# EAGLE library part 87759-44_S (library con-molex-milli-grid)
HEADER
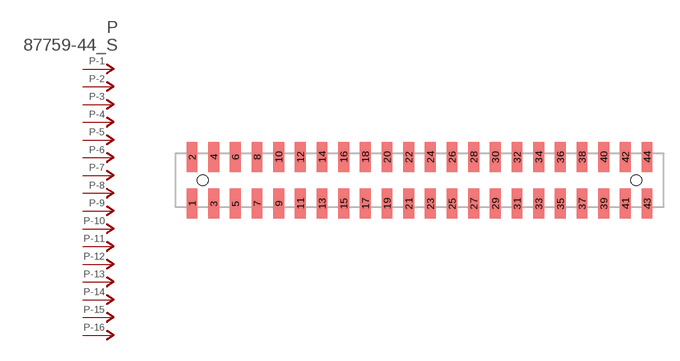
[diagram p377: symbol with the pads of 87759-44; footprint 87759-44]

Designator prefix P; gates -1=P-NV -2=P-N -3=P-N -4=P-N -5=P-N -6=P-N -7=P-N -8=P-N -9=P-N -10=P-N -11=P-N -12=P-N -13=P-N -14=P-N -15=P-N -16=P-N -17=P-N -18=P-N -19=P-N -20=P-N -21=P-N -22=P-N -23=P-N -24=P-N -25=P-N -26=P-N -27=P-N -28=P-N -29=P-N -30=P-N -31=P-N -32=P-N -33=P-N -34=P-N -35=P-N -36=P-N -37=P-N -38=P-N -39=P-N -40=P-N -41=P-N -42=P-N -43=P-N -44=P-N

## 87759-44_S  [87759-44]
1  -1:P  pas
2  -2:P  pas
3  -3:P  pas
4  -4:P  pas
5  -5:P  pas
6  -6:P  pas
7  -7:P  pas
8  -8:P  pas
9  -9:P  pas
10  -10:P  pas
11  -11:P  pas
12  -12:P  pas
13  -13:P  pas
14  -14:P  pas
15  -15:P  pas
16  -16:P  pas
17  -17:P  pas
18  -18:P  pas
19  -19:P  pas
20  -20:P  pas
21  -21:P  pas
22  -22:P  pas
23  -23:P  pas
24  -24:P  pas
25  -25:P  pas
26  -26:P  pas
27  -27:P  pas
28  -28:P  pas
29  -29:P  pas
30  -30:P  pas
31  -31:P  pas
32  -32:P  pas
33  -33:P  pas
34  -34:P  pas
35  -35:P  pas
36  -36:P  pas
37  -37:P  pas
38  -38:P  pas
39  -39:P  pas
40  -40:P  pas
41  -41:P  pas
42  -42:P  pas
43  -43:P  pas
44  -44:P  pas

## Footprint 87759-44 (pad centres in mm)
HEADER SMD Dual Row, Vertical
smd 1 x 2.75: 1 -21,-2.15; 2 -21,2.15; 3 -19,-2.15; 4 -19,2.15; 5 -17,-2.15; 6 -17,2.15; 7 -15,-2.15; 8 -15,2.15; 9 -13,-2.15; 10 -13,2.15; 11 -11,-2.15; 12 -11,2.15; 13 -9,-2.15; 14 -9,2.15; 15 -7,-2.15; 16 -7,2.15; 17 -5,-2.15; 18 -5,2.15; 19 -3,-2.15; 20 -3,2.15; 21 -1,-2.15; 22 -1,2.15; 23 1,-2.15; 24 1,2.15; 25 3,-2.15; 26 3,2.15; 27 5,-2.15; 28 5,2.15; 29 7,-2.15; 30 7,2.15; 31 9,-2.15; 32 9,2.15; 33 11,-2.15; 34 11,2.15; 35 13,-2.15; 36 13,2.15; 37 15,-2.15; 38 15,2.15; 39 17,-2.15; 40 17,2.15; 41 19,-2.15; 42 19,2.15; 43 21,-2.15; 44 21,2.15
hole 1 at -20,0
hole 1 at 20,0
